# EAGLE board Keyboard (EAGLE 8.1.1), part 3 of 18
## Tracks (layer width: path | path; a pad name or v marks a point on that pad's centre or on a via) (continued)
S$1920 (continued)
  Bottom 0: 34.14,81.78 34.07,81.77
S$1921
  Bottom 0: 34.07,81.77 34,81.75
S$1922
  Bottom 0: 34,81.75 33.94,81.73
S$1923
  Bottom 0: 33.94,81.73 33.88,81.69
S$1924
  Bottom 0: 33.88,81.69 33.83,81.65
S$1925
  Bottom 0: 33.83,81.65 31.29,79.12
S$1926
  Bottom 0: 31.29,79.12 25.38,79.12
S$1927
  Bottom 0: 25.38,79.12 25.29,79.35
S$1928
  Bottom 0: 25.29,79.35 25.08,79.63
S$1929
  Bottom 0: 25.08,79.63 24.81,79.86
S$1930
  Bottom 0: 24.81,79.86 24.5,80.01
S$1931
  Bottom 0: 24.5,80.01 24.15,80.07
S$1932
  Bottom 0: 24.15,80.07 23.85,80.05
S$1933
  Bottom 0: 23.85,80.05 24.57,80.78
S$1934
  Bottom 0: 24.57,80.78 29.1,80.78
S$1935
  Bottom 0: 29.1,80.78 29.12,80.7
S$1936
  Bottom 0: 29.12,80.7 29.29,80.39
S$1937
  Bottom 0: 29.29,80.39 29.53,80.14
S$1938
  Bottom 0: 29.53,80.14 29.82,79.95
S$1939
  Bottom 0: 29.82,79.95 30.15,79.84
S$1940
  Bottom 0: 30.15,79.84 30.5,79.83
S$1941
  Bottom 0: 30.5,79.83 30.85,79.89
S$1942
  Bottom 0: 30.85,79.89 31.16,80.04
S$1943
  Bottom 0: 31.16,80.04 31.43,80.26
S$1944
  Bottom 0: 31.43,80.26 31.64,80.55
S$1945
  Bottom 0: 31.64,80.55 31.77,80.87
S$1946
  Bottom 0: 31.77,80.87 31.81,81.22
S$1947
  Bottom 0: 31.81,81.22 31.77,81.56
S$1948
  Bottom 0: 31.77,81.56 31.64,81.89
S$1949
  Bottom 0: 31.64,81.89 31.43,82.17
S$1950
  Bottom 0: 31.43,82.17 31.16,82.39
S$1951
  Bottom 0: 31.16,82.39 30.85,82.55
S$1952
  Bottom 0: 30.85,82.55 30.5,82.61
S$1953
  Bottom 0: 30.5,82.61 30.15,82.59
S$1954
  Bottom 0: 30.15,82.59 29.82,82.48
S$1955
  Bottom 0: 29.82,82.48 29.53,82.29
S$1956
  Bottom 0: 29.53,82.29 29.29,82.04
S$1957
  Bottom 0: 29.29,82.04 29.12,81.73
S$1958
  Bottom 0: 29.12,81.73 29.1,81.66
S$1959
  Bottom 0: 29.1,81.66 27.51,81.66
S$1960
  Bottom 0: 27.51,81.66 27.88,81.86
S$1961
  Bottom 0: 27.88,81.86 28.22,82.14
S$1962
  Bottom 0: 28.22,82.14 28.51,82.49
S$1963
  Bottom 0: 28.51,82.49 28.72,82.88
S$1964
  Bottom 0: 28.72,82.88 28.85,83.31
S$1965
  Bottom 0: 28.85,83.31 28.89,83.76
S$1966
  Bottom 0: 28.89,83.76 28.85,84.2
S$1967
  Bottom 0: 28.85,84.2 28.72,84.63
S$1968
  Bottom 0: 28.72,84.63 28.51,85.03
S$1969
  Bottom 0: 28.51,85.03 28.22,85.37
S$1970
  Bottom 0: 28.22,85.37 27.88,85.66
S$1971
  Bottom 0: 27.88,85.66 27.48,85.87
S$1972
  Bottom 0: 27.48,85.87 27.05,86
S$1973
  Bottom 0: 27.05,86 26.61,86.04
S$1974
  Bottom 0: 26.61,86.04 26.16,86
S$1975
  Bottom 0: 26.16,86 25.73,85.87
S$1976
  Bottom 0: 25.73,85.87 25.34,85.66
S$1977
  Bottom 0: 25.34,85.66 24.99,85.37
S$1978
  Bottom 0: 24.99,85.37 24.7,85.03
S$1979
  Bottom 0: 24.7,85.03 24.49,84.63
S$1980
  Bottom 0: 24.49,84.63 24.37,84.2
S$1981
  Bottom 0: 24.37,84.2 24.32,83.76
S$1982
  Bottom 0: 24.32,83.76 24.37,83.31
S$1983
  Bottom 0: 24.37,83.31 24.49,82.88
S$1984
  Bottom 0: 24.49,82.88 24.7,82.49
S$1985
  Bottom 0: 24.7,82.49 24.99,82.14
S$1986
  Bottom 0: 24.99,82.14 25.34,81.86
S$1987
  Bottom 0: 25.34,81.86 25.7,81.66
S$1988
  Bottom 0: 25.7,81.66 24.39,81.66
S$1989
  Bottom 0: 24.39,81.66 24.32,81.65
S$1990
  Bottom 0: 24.32,81.65 24.25,81.64
S$1991
  Bottom 0: 24.25,81.64 24.19,81.61
S$1992
  Bottom 0: 24.19,81.61 24.13,81.57
S$1993
  Bottom 0: 24.13,81.57 24.07,81.53
S$1994
  Bottom 0: 24.07,81.53 22.24,79.7
S$1995
  Bottom 0: 22.24,79.7 22.24,80.54
S$1996
  Bottom 0: 22.24,80.54 22.31,80.61
S$1997
  Bottom 0: 22.31,80.61 22.36,80.61
S$1998
  Bottom 0: 22.36,80.61 22.5,80.63
S$1999
  Bottom 0: 22.5,80.63 22.62,80.69
S$2000
  Bottom 0: 22.62,80.69 22.71,80.79
S$2001
  Bottom 0: 22.71,80.79 22.78,80.91
S$2002
  Bottom 0: 22.78,80.91 22.8,81.05
S$2003
  Bottom 0: 22.8,81.05 22.8,84.4
S$2004
  Bottom 0: 22.8,84.4 25.65,87.25
S$2005
  Bottom 0: 25.65,87.25 25.69,87.32
S$2006
  Bottom 0: 25.69,87.32 25.72,87.35
S$2007
  Bottom 0: 25.72,87.35 25.73,87.39
S$2008
  Bottom 0: 25.73,87.39 25.76,87.45
S$2009
  Bottom 0: 25.76,87.45 25.76,87.51
S$2010
  Bottom 0: 25.76,87.51 25.78,87.57
S$2011
  Bottom 0: 25.78,87.57 25.78,87.69
S$2012
  Bottom 0: 25.78,87.69 26.23,87.69
S$2013
  Bottom 0: 26.23,87.69 26.3,87.7
S$2014
  Bottom 0: 26.3,87.7 26.37,87.74
S$2015
  Bottom 0: 26.37,87.74 26.43,87.8
S$2016
  Bottom 0: 26.43,87.8 26.47,87.87
S$2017
  Bottom 0: 26.47,87.87 26.48,87.95
S$2018
  Bottom 0: 26.48,87.95 26.48,89.72
S$2019
  Bottom 0: 26.48,89.72 26.47,89.8
S$2020
  Bottom 0: 26.47,89.8 26.43,89.87
S$2021
  Bottom 0: 26.43,89.87 26.37,89.93
S$2022
  Bottom 0: 26.37,89.93 26.3,89.97
S$2023
  Bottom 0: 26.3,89.97 26.23,89.98
S$2024
  Bottom 0: 26.23,89.98 24.45,89.98
S$2025
  Bottom 0: 24.45,89.98 24.37,89.97
S$2026
  Bottom 0: 24.37,89.97 24.3,89.93
S$2027
  Bottom 0: 24.3,89.93 24.24,89.87
S$2028
  Bottom 0: 24.24,89.87 24.2,89.8
S$2029
  Bottom 0: 24.2,89.8 24.19,89.72
S$2030
  Bottom 0: 24.19,89.72 24.19,87.95
S$2031
  Bottom 0: 24.19,87.95 24.2,87.87
S$2032
  Bottom 0: 24.2,87.87 24.24,87.8
S$2033
  Bottom 0: 24.24,87.8 24.3,87.74
S$2034
  Bottom 0: 24.3,87.74 24.37,87.7
S$2035
  Bottom 0: 24.37,87.7 24.45,87.69
S$2036
  Bottom 0: 24.45,87.69 24.83,87.69
S$2037
  Bottom 0: 24.83,87.69 22.05,84.91
S$2038
  Bottom 0: 22.05,84.91 22,84.85
S$2039
  Bottom 0: 22,84.85 21.96,84.79
S$2040
  Bottom 0: 21.96,84.79 21.94,84.73
S$2041
  Bottom 0: 21.94,84.73 21.92,84.66
S$2042
  Bottom 0: 21.92,84.66 21.92,84.59
S$2043
  Bottom 0: 21.92,84.59 21.92,81.44
S$2044
  Bottom 0: 21.92,81.44 21.87,81.41
S$2045
  Bottom 0: 21.87,81.41 21.82,81.36
S$2046
  Bottom 0: 21.82,81.36 21.49,81.04
S$2047
  Bottom 0: 21.49,81.04 21.45,80.99
S$2048
  Bottom 0: 21.45,80.99 21.41,80.93
S$2049
  Bottom 0: 21.41,80.93 21.38,80.86
S$2050
  Bottom 0: 21.38,80.86 21.36,80.8
S$2051
  Bottom 0: 21.36,80.8 21.36,80.72
S$2052
  Bottom 0: 21.36,80.72 21.36,76.79
S$2053
  Bottom 0: 21.36,76.79 21.36,76.72
S$2054
  Bottom 0: 21.36,76.72 21.38,76.65
S$2055
  Bottom 0: 21.38,76.65 21.4,76.59
S$2056
  Bottom 0: 21.4,76.59 21.45,76.53
S$2057
  Bottom 0: 21.45,76.53 21.48,76.47
S$2058
  Bottom 0: 21.48,76.47 21.84,76.12
S$2059
  Bottom 0: 21.84,76.12 21.7,75.89
S$2060
  Bottom 0: 21.7,75.89 21.61,75.58
S$2061
  Bottom 0: 21.61,75.58 21.61,75.26
S$2062
  Bottom 0: 21.61,75.26 21.7,74.94
S$2063
  Bottom 0: 21.7,74.94 21.87,74.67
S$2064
  Bottom 0: 21.87,74.67 22.1,74.44
S$2065
  Bottom 0: 22.1,74.44 22.39,74.3
S$2066
  Bottom 0: 22.39,74.3 22.71,74.23
S$2067
  Bottom 0: 22.71,74.23 23.04,74.25
S$2068
  Bottom 0: 23.04,74.25 23.34,74.36
S$2069
  Bottom 0: 23.34,74.36 23.61,74.55
S$2070
  Bottom 0: 23.61,74.55 23.82,74.8
S$2071
  Bottom 0: 23.82,74.8 23.94,75.1
S$2072
  Bottom 0: 23.94,75.1 23.99,75.42
S$2073
  Bottom 0: 23.99,75.42 23.94,75.74
S$2074
  Bottom 0: 23.94,75.74 23.9,75.85
S$2075
  Bottom 0: 23.9,75.85 24.7,75.05
S$2076
  Bottom 0: 24.7,75.05 24.7,68.48
S$2077
  Bottom 0: 24.7,68.48 24.7,68.4
S$2078
  Bottom 0: 24.7,68.4 24.72,68.34
S$2079
  Bottom 0: 24.72,68.34 24.74,68.28
S$2080
  Bottom 0: 24.74,68.28 24.78,68.21
S$2081
  Bottom 0: 24.78,68.21 24.82,68.17
S$2082
  Bottom 0: 24.82,68.17 29.65,63.33
S$2083
  Bottom 0: 29.65,63.33 29.71,63.29
S$2084
  Bottom 0: 29.71,63.29 23.49,63.29
S$2085
  Bottom 0: 23.49,63.29 23.49,69.53
S$2086
  Bottom 0: 23.49,69.53 23.49,69.6
S$2087
  Bottom 0: 23.49,69.6 23.47,69.67
S$2088
  Bottom 0: 23.47,69.67 23.45,69.73
S$2089
  Bottom 0: 23.45,69.73 23.4,69.79
S$2090
  Bottom 0: 23.4,69.79 23.36,69.85
S$2091
  Bottom 0: 23.36,69.85 12.61,80.6
S$2092
  Bottom 0: 12.61,80.6 12.71,80.87
S$2093
  Bottom 0: 12.71,80.87 12.76,81.22
S$2094
  Bottom 0: 12.76,81.22 12.71,81.56
S$2095
  Bottom 0: 12.71,81.56 12.59,81.89
S$2096
  Bottom 0: 12.59,81.89 12.38,82.17
S$2097
  Bottom 0: 12.38,82.17 12.11,82.39
S$2098
  Bottom 0: 12.11,82.39 11.8,82.55
S$2099
  Bottom 0: 11.8,82.55 11.45,82.61
S$2100
  Bottom 0: 11.45,82.61 11.1,82.59
S$2101
  Bottom 0: 11.1,82.59 10.77,82.48
S$2102
  Bottom 0: 10.77,82.48 10.48,82.29
S$2103
  Bottom 0: 10.48,82.29 10.29,82.1
S$2104
  Bottom 0: 10.29,82.1 10.29,82.12
S$2105
  Bottom 0: 10.29,82.12 10.49,82.31
S$2106
  Bottom 0: 10.49,82.31 10.55,82.38
S$2107
  Bottom 0: 10.55,82.38 10.59,82.45
S$2108
  Bottom 0: 10.59,82.45 10.63,82.53
S$2109
  Bottom 0: 10.63,82.53 10.65,82.62
S$2110
  Bottom 0: 10.65,82.62 10.65,82.71
S$2111
  Bottom 0: 10.65,82.71 10.65,87.58
S$2112
  Bottom 0: 10.65,87.58 10.65,87.67
S$2113
  Bottom 0: 10.65,87.67 10.63,87.75
S$2114
  Bottom 0: 10.63,87.75 10.59,87.84
S$2115
  Bottom 0: 10.59,87.84 10.55,87.91
S$2116
  Bottom 0: 10.55,87.91 10.49,87.98
S$2117
  Bottom 0: 10.49,87.98 9.93,88.54
S$2118
  Bottom 0: 9.93,88.54 9.97,88.84
S$2119
  Bottom 0: 9.97,88.84 9.92,89.16
S$2120
  Bottom 0: 9.92,89.16 9.78,89.46
S$2121
  Bottom 0: 9.78,89.46 9.57,89.7
S$2122
  Bottom 0: 9.57,89.7 9.3,89.88
S$2123
  Bottom 0: 9.3,89.88 8.99,89.97
S$2124
  Bottom 0: 8.99,89.97 8.66,89.97
S$2125
  Bottom 0: 8.66,89.97 8.35,89.88
S$2126
  Bottom 0: 8.35,89.88 8.08,89.7
S$2127
  Bottom 0: 8.08,89.7 7.87,89.46
S$2128
  Bottom 0: 7.87,89.46 7.73,89.16
S$2129
  Bottom 0: 7.73,89.16 7.68,88.84
S$2130
  Bottom 0: 7.68,88.84 7.73,88.52
S$2131
  Bottom 0: 7.73,88.52 7.87,88.22
S$2132
  Bottom 0: 7.87,88.22 8.08,87.97
S$2133
  Bottom 0: 8.08,87.97 8.35,87.8
S$2134
  Bottom 0: 8.35,87.8 8.66,87.7
S$2135
  Bottom 0: 8.66,87.7 8.99,87.7
S$2136
  Bottom 0: 8.99,87.7 9.11,87.74
S$2137
  Bottom 0: 9.11,87.74 9.52,87.34
S$2138
  Bottom 0: 9.52,87.34 9.52,84.92
S$2139
  Bottom 0: 9.52,84.92 9.46,85.03
S$2140
  Bottom 0: 9.46,85.03 9.17,85.37
S$2141
  Bottom 0: 9.17,85.37 8.83,85.66
S$2142
  Bottom 0: 8.83,85.66 8.43,85.87
S$2143
  Bottom 0: 8.43,85.87 8,86
S$2144
  Bottom 0: 8,86 7.56,86.04
S$2145
  Bottom 0: 7.56,86.04 7.11,86
S$2146
  Bottom 0: 7.11,86 6.68,85.87
S$2147
  Bottom 0: 6.68,85.87 6.29,85.66
S$2148
  Bottom 0: 6.29,85.66 5.94,85.37
S$2149
  Bottom 0: 5.94,85.37 5.65,85.03
S$2150
  Bottom 0: 5.65,85.03 5.44,84.63
S$2151
  Bottom 0: 5.44,84.63 5.32,84.2
S$2152
  Bottom 0: 5.32,84.2 5.27,83.76
S$2153
  Bottom 0: 5.27,83.76 5.32,83.31
S$2154
  Bottom 0: 5.32,83.31 5.44,82.88
S$2155
  Bottom 0: 5.44,82.88 5.65,82.49
S$2156
  Bottom 0: 5.65,82.49 5.94,82.14
S$2157
  Bottom 0: 5.94,82.14 6.29,81.86
S$2158
  Bottom 0: 6.29,81.86 6.68,81.64
S$2159
  Bottom 0: 6.68,81.64 7.11,81.52
S$2160
  Bottom 0: 7.11,81.52 7.56,81.47
S$2161
  Bottom 0: 7.56,81.47 8,81.52
S$2162
  Bottom 0: 8,81.52 8.43,81.64
S$2163
  Bottom 0: 8.43,81.64 8.83,81.86
S$2164
  Bottom 0: 8.83,81.86 9.16,82.13
S$2165
  Bottom 0: 9.16,82.13 9.16,74.32
S$2166
  Bottom 0: 9.16,74.32 9.16,74.23
S$2167
  Bottom 0: 9.16,74.23 9.18,74.14
S$2168
  Bottom 0: 9.18,74.14 9.22,74.06
S$2169
  Bottom 0: 9.22,74.06 9.26,73.98
S$2170
  Bottom 0: 9.26,73.98 9.32,73.92
S$2171
  Bottom 0: 9.32,73.92 12.72,70.51
S$2172
  Bottom 0: 12.72,70.51 12.62,70.41
S$2173
  Bottom 0: 12.62,70.41 12.49,70.11
S$2174
  Bottom 0: 12.49,70.11 12.44,69.79
S$2175
  Bottom 0: 12.44,69.79 12.49,69.47
S$2176
  Bottom 0: 12.49,69.47 12.62,69.16
S$2177
  Bottom 0: 12.62,69.16 12.84,68.92
S$2178
  Bottom 0: 12.84,68.92 13.11,68.75
S$2179
  Bottom 0: 13.11,68.75 13.42,68.65
S$2180
  Bottom 0: 13.42,68.65 13.75,68.65
S$2181
  Bottom 0: 13.75,68.65 14.06,68.75
S$2182
  Bottom 0: 14.06,68.75 14.33,68.92
S$2183
  Bottom 0: 14.33,68.92 14.54,69.16
S$2184
  Bottom 0: 14.54,69.16 14.68,69.47
S$2185
  Bottom 0: 14.68,69.47 14.73,69.79
S$2186
  Bottom 0: 14.73,69.79 14.68,70.11
S$2187
  Bottom 0: 14.68,70.11 14.54,70.41
S$2188
  Bottom 0: 14.54,70.41 14.33,70.65
S$2189
  Bottom 0: 14.33,70.65 14.06,70.83
S$2190
  Bottom 0: 14.06,70.83 13.99,70.85
S$2191
  Bottom 0: 13.99,70.85 13.98,70.85
S$2192
  Bottom 0: 13.98,70.85 10.29,74.55
S$2193
  Bottom 0: 10.29,74.55 10.29,74.9
S$2194
  Bottom 0: 10.29,74.9 10.44,74.66
S$2195
  Bottom 0: 10.44,74.66 10.67,74.44
S$2196
  Bottom 0: 10.67,74.44 10.96,74.29
S$2197
  Bottom 0: 10.96,74.29 11.29,74.23
S$2198
  Bottom 0: 11.29,74.23 11.61,74.24
S$2199
  Bottom 0: 11.61,74.24 11.7,74.28
S$2200
  Bottom 0: 11.7,74.28 13.34,72.64
S$2201
  Bottom 0: 13.34,72.64 13.4,72.58
S$2202
  Bottom 0: 13.4,72.58 13.48,72.53
S$2203
  Bottom 0: 13.48,72.53 13.56,72.5
S$2204
  Bottom 0: 13.56,72.5 13.65,72.48
S$2205
  Bottom 0: 13.65,72.48 13.74,72.47
S$2206
  Bottom 0: 13.74,72.47 15.09,72.47
S$2207
  Bottom 0: 15.09,72.47 15.21,72.29
S$2208
  Bottom 0: 15.21,72.29 15.44,72.07
S$2209
  Bottom 0: 15.44,72.07 15.56,72.01
S$2210
  Bottom 0: 15.56,72.01 15.56,65.05
S$2211
  Bottom 0: 15.56,65.05 14.46,63.95
S$2212
  Bottom 0: 14.46,63.95 14.56,64.26
S$2213
  Bottom 0: 14.56,64.26 14.6,64.71
S$2214
  Bottom 0: 14.6,64.71 14.56,65.15
S$2215
  Bottom 0: 14.56,65.15 14.43,65.58
S$2216
  Bottom 0: 14.43,65.58 14.22,65.98
S$2217
  Bottom 0: 14.22,65.98 13.93,66.32
S$2218
  Bottom 0: 13.93,66.32 13.59,66.61
S$2219
  Bottom 0: 13.59,66.61 13.19,66.82
S$2220
  Bottom 0: 13.19,66.82 12.76,66.94
S$2221
  Bottom 0: 12.76,66.94 12.32,66.99
S$2222
  Bottom 0: 12.32,66.99 11.87,66.94
S$2223
  Bottom 0: 11.87,66.94 11.44,66.82
S$2224
  Bottom 0: 11.44,66.82 11.05,66.61
S$2225
  Bottom 0: 11.05,66.61 10.7,66.32
S$2226
  Bottom 0: 10.7,66.32 10.41,65.98
S$2227
  Bottom 0: 10.41,65.98 10.2,65.58
S$2228
  Bottom 0: 10.2,65.58 10.08,65.15
S$2229
  Bottom 0: 10.08,65.15 10.03,64.71
S$2230
  Bottom 0: 10.03,64.71 10.08,64.26
S$2231
  Bottom 0: 10.08,64.26 10.2,63.83
S$2232
  Bottom 0: 10.2,63.83 10.41,63.44
S$2233
  Bottom 0: 10.41,63.44 10.7,63.09
S$2234
  Bottom 0: 10.7,63.09 11.05,62.81
S$2235
  Bottom 0: 11.05,62.81 11.44,62.59
S$2236
  Bottom 0: 11.44,62.59 11.87,62.47
S$2237
  Bottom 0: 11.87,62.47 12.32,62.42
S$2238
  Bottom 0: 12.32,62.42 12.76,62.47
S$2239
  Bottom 0: 12.76,62.47 13.07,62.56
S$2240
  Bottom 0: 13.07,62.56 11.64,61.13
S$2241
  Bottom 0: 11.64,61.13 11.58,61.06
S$2242
  Bottom 0: 11.58,61.06 11.53,60.99
S$2243
  Bottom 0: 11.53,60.99 11.5,60.91
S$2244
  Bottom 0: 11.5,60.91 11.48,60.82
S$2245
  Bottom 0: 11.48,60.82 11.47,60.73
S$2246
  Bottom 0: 11.47,60.73 11.47,49.4
S$2247
  Bottom 0: 11.47,49.4 11.48,49.32
S$2248
  Bottom 0: 11.48,49.32 1.2,39.04
S$2249
  Bottom 0: 1.2,39.04 1.14,38.98
S$2250
  Bottom 0: 1.14,38.98 1.09,38.9
S$2251
  Bottom 0: 1.09,38.9 1.06,38.82
S$2252
  Bottom 0: 1.06,38.82 1.04,38.73
S$2253
  Bottom 0: 1.04,38.73 1.03,38.64
S$2254
  Bottom 0: 1.03,38.64 1.03,14.78
S$2255
  Bottom 0: 1.03,14.78 0.91,14.71
S$2256
  Bottom 0: 0.91,14.71 0.68,14.49
S$2257
  Bottom 0: 0.68,14.49 0.51,14.22
S$2258
  Bottom 0: 0.51,14.22 0.42,13.9
S$2259
  Bottom 0: 0.42,13.9 0.42,13.58
S$2260
  Bottom 0: 0.42,13.58 0.51,13.26
S$2261
  Bottom 0: 0.51,13.26 0.68,12.99
S$2262
  Bottom 0: 0.68,12.99 0.91,12.76
S$2263
  Bottom 0: 0.91,12.76 1.2,12.62
S$2264
  Bottom 0: 1.2,12.62 1.52,12.55
S$2265
  Bottom 0: 1.52,12.55 1.84,12.57
S$2266
  Bottom 0: 1.84,12.57 2.15,12.68
S$2267
  Bottom 0: 2.15,12.68 2.41,12.87
S$2268
  Bottom 0: 2.41,12.87 2.62,13.12
S$2269
  Bottom 0: 2.62,13.12 2.75,13.42
S$2270
  Bottom 0: 2.75,13.42 2.79,13.74
S$2271
  Bottom 0: 2.79,13.74 2.75,14.06
S$2272
  Bottom 0: 2.75,14.06 2.62,14.36
S$2273
  Bottom 0: 2.62,14.36 2.41,14.61
S$2274
  Bottom 0: 2.41,14.61 2.17,14.79
S$2275
  Bottom 0: 2.17,14.79 2.17,38.41
S$2276
  Bottom 0: 2.17,38.41 12.43,48.67
S$2277
  Bottom 0: 12.43,48.67 16.34,48.67
S$2278
  Bottom 0: 16.34,48.67 19.68,45.32
S$2279
  Bottom 0: 19.68,45.32 19.68,43.85
S$2280
  Bottom 0: 19.68,43.85 19.52,44.07
S$2281
  Bottom 0: 19.52,44.07 19.26,44.3
S$2282
  Bottom 0: 19.26,44.3 18.94,44.45
S$2283
  Bottom 0: 18.94,44.45 18.59,44.51
S$2284
  Bottom 0: 18.59,44.51 18.24,44.49
S$2285
  Bottom 0: 18.24,44.49 17.91,44.38
S$2286
  Bottom 0: 17.91,44.38 17.62,44.19
S$2287
  Bottom 0: 17.62,44.19 17.38,43.94
S$2288
  Bottom 0: 17.38,43.94 17.21,43.63
S$2289
  Bottom 0: 17.21,43.63 17.12,43.29
S$2290
  Bottom 0: 17.12,43.29 17.12,42.94
S$2291
  Bottom 0: 17.12,42.94 17.21,42.6
S$2292
  Bottom 0: 17.21,42.6 17.26,42.5
S$2293
  Bottom 0: 17.26,42.5 9.61,34.85
S$2294
  Bottom 0: 9.61,34.85 9.53,34.74
S$2295
  Bottom 0: 9.53,34.74 9.5,34.67
S$2296
  Bottom 0: 9.5,34.67 9.49,34.61
S$2297
  Bottom 0: 9.49,34.61 9.48,34.54
S$2298
  Bottom 0: 9.48,34.54 9.48,13.78
S$2299
  Bottom 0: 9.48,13.78 7.78,13.78
S$2300
  Bottom 0: 7.78,13.78 7.7,13.77
S$2301
  Bottom 0: 7.7,13.77 7.63,13.73
S$2302
  Bottom 0: 7.63,13.73 7.57,13.67
S$2303
  Bottom 0: 7.57,13.67 7.54,13.6
S$2304
  Bottom 0: 7.54,13.6 7.52,13.53
S$2305
  Bottom 0: 7.52,13.53 7.52,13.08
S$2306
  Bottom 0: 7.52,13.08 7.4,13.08
S$2307
  Bottom 0: 7.4,13.08 7.18,13.02
S$2308
  Bottom 0: 7.18,13.02 7.01,12.86
S$2309
  Bottom 0: 7.01,12.86 6.96,12.64
S$2310
  Bottom 0: 6.96,12.64 6.96,12.1
S$2311
  Bottom 0: 6.96,12.1 2.06,7.21
S$2312
  Bottom 0: 2.06,7.21 1.84,7.29
S$2313
  Bottom 0: 1.84,7.29 1.52,7.31
S$2314
  Bottom 0: 1.52,7.31 1.2,7.24
S$2315
  Bottom 0: 1.2,7.24 0.91,7.09
S$2316
  Bottom 0: 0.91,7.09 0.68,6.87
S$2317
  Bottom 0: 0.68,6.87 0.51,6.6
S$2318
  Bottom 0: 0.51,6.6 0.42,6.28
S$2319
  Bottom 0: 0.42,6.28 0.42,5.96
S$2320
  Bottom 0: 0.42,5.96 0.51,5.64
S$2321
  Bottom 0: 0.51,5.64 0.68,5.37
S$2322
  Bottom 0: 0.68,5.37 0.91,5.14
S$2323
  Bottom 0: 0.91,5.14 1.2,5
S$2324
  Bottom 0: 1.2,5 1.52,4.93
S$2325
  Bottom 0: 1.52,4.93 1.84,4.95
S$2326
  Bottom 0: 1.84,4.95 2.15,5.06
S$2327
  Bottom 0: 2.15,5.06 2.41,5.25
S$2328
  Bottom 0: 2.41,5.25 2.62,5.5
S$2329
  Bottom 0: 2.62,5.5 2.75,5.8
S$2330
  Bottom 0: 2.75,5.8 2.79,6.12
S$2331
  Bottom 0: 2.79,6.12 2.75,6.44
S$2332
  Bottom 0: 2.75,6.44 2.69,6.58
S$2333
  Bottom 0: 2.69,6.58 7.65,11.53
S$2334
  Bottom 0: 7.65,11.53 7.7,11.5
S$2335
  Bottom 0: 7.7,11.5 7.78,11.49
S$2336
  Bottom 0: 7.78,11.49 9.48,11.49
S$2337
  Bottom 0: 9.48,11.49 9.48,10.99
S$2338
  Bottom 0: 9.48,10.99 9.49,10.91
S$2339
  Bottom 0: 9.49,10.91 9.5,10.85
S$2340
  Bottom 0: 9.5,10.85 9.53,10.79
S$2341
  Bottom 0: 9.53,10.79 9.57,10.73
S$2342
  Bottom 0: 9.57,10.73 9.61,10.67
S$2343
  Bottom 0: 9.61,10.67 10.52,9.76
S$2344
  Bottom 0: 10.52,9.76 10.38,9.8
S$2345
  Bottom 0: 10.38,9.8 9.94,9.84
S$2346
  Bottom 0: 9.94,9.84 9.49,9.8
S$2347
  Bottom 0: 9.49,9.8 9.06,9.67
S$2348
  Bottom 0: 9.06,9.67 8.67,9.46
S$2349
  Bottom 0: 8.67,9.46 8.32,9.17
S$2350
  Bottom 0: 8.32,9.17 8.04,8.83
S$2351
  Bottom 0: 8.04,8.83 7.83,8.43
S$2352
  Bottom 0: 7.83,8.43 7.7,8
S$2353
  Bottom 0: 7.7,8 7.65,7.56
S$2354
  Bottom 0: 7.65,7.56 7.7,7.11
S$2355
  Bottom 0: 7.7,7.11 7.83,6.68
S$2356
  Bottom 0: 7.83,6.68 8.04,6.29
S$2357
  Bottom 0: 8.04,6.29 8.32,5.94
S$2358
  Bottom 0: 8.32,5.94 8.67,5.66
S$2359
  Bottom 0: 8.67,5.66 9.06,5.44
S$2360
  Bottom 0: 9.06,5.44 9.49,5.32
S$2361
  Bottom 0: 9.49,5.32 9.94,5.27
S$2362
  Bottom 0: 9.94,5.27 10.38,5.32
S$2363
  Bottom 0: 10.38,5.32 10.81,5.44
S$2364
  Bottom 0: 10.81,5.44 11.21,5.66
S$2365
  Bottom 0: 11.21,5.66 11.55,5.94
S$2366
  Bottom 0: 11.55,5.94 11.84,6.29
S$2367
  Bottom 0: 11.84,6.29 12.05,6.68
S$2368
  Bottom 0: 12.05,6.68 12.18,7.11
S$2369
  Bottom 0: 12.18,7.11 12.22,7.56
S$2370
  Bottom 0: 12.22,7.56 12.18,8
S$2371
  Bottom 0: 12.18,8 12.14,8.14
S$2372
  Bottom 0: 12.14,8.14 13.88,6.4
S$2373
  Bottom 0: 13.88,6.4 13.84,6.41
S$2374
  Bottom 0: 13.84,6.41 13.48,6.39
S$2375
  Bottom 0: 13.48,6.39 13.15,6.28
S$2376
  Bottom 0: 13.15,6.28 12.86,6.09
S$2377
  Bottom 0: 12.86,6.09 12.62,5.84
S$2378
  Bottom 0: 12.62,5.84 12.45,5.53
S$2379
  Bottom 0: 12.45,5.53 12.36,5.19
S$2380
  Bottom 0: 12.36,5.19 12.36,4.84
S$2381
  Bottom 0: 12.36,4.84 12.45,4.5
S$2382
  Bottom 0: 12.45,4.5 12.62,4.19
S$2383
  Bottom 0: 12.62,4.19 12.86,3.94
S$2384
  Bottom 0: 12.86,3.94 13.15,3.75
S$2385
  Bottom 0: 13.15,3.75 13.48,3.65
S$2386
  Bottom 0: 13.48,3.65 13.84,3.62
S$2387
  Bottom 0: 13.84,3.62 14.18,3.69
S$2388
  Bottom 0: 14.18,3.69 14.49,3.84
S$2389
  Bottom 0: 14.49,3.84 14.77,4.06
S$2390
  Bottom 0: 14.77,4.06 14.97,4.35
S$2391
  Bottom 0: 14.97,4.35 15.1,4.67
S$2392
  Bottom 0: 15.1,4.67 15.15,5.02
S$2393
  Bottom 0: 15.15,5.02 15.13,5.15
S$2394
  Bottom 0: 15.13,5.15 16.04,4.24
S$2395
  Bottom 0: 16.04,4.24 16.04,2.29
S$2396
  Bottom 0: 16.04,2.29 16.05,2.22
S$2397
  Bottom 0: 16.05,2.22 16.06,2.15
S$2398
  Bottom 0: 16.06,2.15 16.08,2.09
S$2399
  Bottom 0: 16.08,2.09 16.13,2.03
S$2400
  Bottom 0: 16.13,2.03 16.16,1.97
S$2401
  Bottom 0: 16.16,1.97 16.71,1.43
S$2402
  Bottom 0: 16.71,1.43 9.06,1.43
S$2403
  Bottom 0: 9.06,1.43 8.64,1.86
S$2404
  Bottom 0: 8.64,1.86 8.75,2.13
S$2405
  Bottom 0: 8.75,2.13 8.79,2.48
S$2406
  Bottom 0: 8.79,2.48 8.75,2.82
S$2407
  Bottom 0: 8.75,2.82 8.62,3.15
S$2408
  Bottom 0: 8.62,3.15 8.41,3.43
S$2409
  Bottom 0: 8.41,3.43 8.14,3.65
S$2410
  Bottom 0: 8.14,3.65 7.83,3.81
S$2411
  Bottom 0: 7.83,3.81 7.49,3.87
S$2412
  Bottom 0: 7.49,3.87 7.13,3.85
S$2413
  Bottom 0: 7.13,3.85 6.8,3.74
S$2414
  Bottom 0: 6.8,3.74 6.51,3.55
S$2415
  Bottom 0: 6.51,3.55 6.27,3.3
S$2416
  Bottom 0: 6.27,3.3 6.1,2.99
S$2417
  Bottom 0: 6.1,2.99 6.01,2.65
S$2418
  Bottom 0: 6.01,2.65 6.01,2.3
S$2419
  Bottom 0: 6.01,2.3 6.1,1.96
S$2420
  Bottom 0: 6.1,1.96 6.27,1.65
S$2421
  Bottom 0: 6.27,1.65 6.51,1.4
S$2422
  Bottom 0: 6.51,1.4 6.8,1.21
S$2423
  Bottom 0: 6.8,1.21 7.13,1.1
S$2424
  Bottom 0: 7.13,1.1 7.49,1.08
S$2425
  Bottom 0: 7.49,1.08 7.83,1.15
S$2426
  Bottom 0: 7.83,1.15 8.01,1.23
S$2427
  Bottom 0: 8.01,1.23 8.57,0.68
S$2428
  Bottom 0: 8.57,0.68 8.62,0.63
S$2429
  Bottom 0: 8.62,0.63 8.68,0.6
S$2430
  Bottom 0: 8.68,0.6 8.74,0.57
S$2431
  Bottom 0: 8.74,0.57 8.81,0.55
S$2432
  Bottom 0: 8.81,0.55 8.88,0.55
S$2433
  Bottom 0: 275.8,1.07 276.1,1.12
S$2434
  Bottom 0: 276.1,1.12 276.21,1.09
S$2435
  Bottom 0: 276.21,1.09 276.56,1.07
S$2436
  Bottom 0: 276.56,1.07 276.9,1.13
S$2437
  Bottom 0: 276.9,1.13 277.22,1.28
S$2438
  Bottom 0: 277.22,1.28 277.49,1.51
S$2439
  Bottom 0: 277.49,1.51 277.7,1.79
S$2440
  Bottom 0: 277.7,1.79 277.82,2.12
S$2441
  Bottom 0: 277.82,2.12 277.87,2.46
S$2442
  Bottom 0: 277.87,2.46 277.82,2.81
S$2443
  Bottom 0: 277.82,2.81 277.7,3.13
S$2444
  Bottom 0: 277.7,3.13 277.49,3.42
S$2445
  Bottom 0: 277.49,3.42 277.22,3.64
S$2446
  Bottom 0: 277.22,3.64 276.9,3.79
S$2447
  Bottom 0: 276.9,3.79 276.56,3.85
S$2448
  Bottom 0: 276.56,3.85 276.21,3.83
S$2449
  Bottom 0: 276.21,3.83 276.1,3.8
S$2450
  Bottom 0: 276.1,3.8 275.8,3.85
S$2451
  Bottom 0: 275.8,3.85 275.44,3.83
S$2452
  Bottom 0: 275.44,3.83 275.12,3.73
S$2453
  Bottom 0: 275.12,3.73 274.82,3.54
S$2454
  Bottom 0: 274.82,3.54 274.58,3.28
S$2455
  Bottom 0: 274.58,3.28 274.41,2.97
S$2456
  Bottom 0: 274.41,2.97 274.39,2.9
S$2457
  Bottom 0: 274.39,2.9 271.22,2.9
S$2458
  Bottom 0: 271.22,2.9 270.47,3.65
S$2459
  Bottom 0: 270.47,3.65 270.49,3.67
S$2460
  Bottom 0: 270.49,3.67 270.54,3.98
S$2461
  Bottom 0: 270.54,3.98 270.49,4.28
S$2462
  Bottom 0: 270.49,4.28 270.36,4.55
S$2463
  Bottom 0: 270.36,4.55 270.15,4.77
S$2464
  Bottom 0: 270.15,4.77 269.89,4.92
S$2465
  Bottom 0: 269.89,4.92 269.6,4.99
S$2466
  Bottom 0: 269.6,4.99 269.29,4.97
S$2467
  Bottom 0: 269.29,4.97 269.01,4.85
S$2468
  Bottom 0: 269.01,4.85 268.77,4.67
S$2469
  Bottom 0: 268.77,4.67 268.61,4.42
S$2470
  Bottom 0: 268.61,4.42 268.52,4.13
S$2471
  Bottom 0: 268.52,4.13 268.52,3.82
S$2472
  Bottom 0: 268.52,3.82 268.61,3.53
S$2473
  Bottom 0: 268.61,3.53 268.77,3.28
S$2474
  Bottom 0: 268.77,3.28 269.01,3.1
S$2475
  Bottom 0: 269.01,3.1 269.29,2.98
S$2476
  Bottom 0: 269.29,2.98 269.6,2.96
S$2477
  Bottom 0: 269.6,2.96 269.85,3.02
S$2478
  Bottom 0: 269.85,3.02 270.72,2.15
S$2479
  Bottom 0: 270.72,2.15 270.78,2.11
S$2480
  Bottom 0: 270.78,2.11 270.84,2.06
S$2481
  Bottom 0: 270.84,2.06 270.9,2.04
S$2482
  Bottom 0: 270.9,2.04 270.96,2.02
S$2483
  Bottom 0: 270.96,2.02 271.04,2.02
S$2484
  Bottom 0: 271.04,2.02 274.39,2.02
S$2485
  Bottom 0: 274.39,2.02 274.41,1.95
S$2486
  Bottom 0: 274.41,1.95 274.58,1.64
S$2487
  Bottom 0: 274.58,1.64 274.82,1.38
S$2488
  Bottom 0: 274.82,1.38 275.12,1.2
S$2489
  Bottom 0: 275.12,1.2 275.44,1.09
S$2490
  Bottom 0: 275.44,1.09 275.8,1.07
S$2491
  Bottom 0: 197.99,1.08 198.33,1.15
S$2492
  Bottom 0: 198.33,1.15 198.65,1.3
S$2493
  Bottom 0: 198.65,1.3 198.91,1.52
S$2494
  Bottom 0: 198.91,1.52 199.12,1.81
S$2495
  Bottom 0: 199.12,1.81 199.25,2.13
S$2496
  Bottom 0: 199.25,2.13 199.3,2.48
S$2497
  Bottom 0: 199.3,2.48 199.25,2.82
S$2498
  Bottom 0: 199.25,2.82 199.12,3.15
S$2499
  Bottom 0: 199.12,3.15 198.91,3.43
S$2500
  Bottom 0: 198.91,3.43 198.65,3.65
S$2501
  Bottom 0: 198.65,3.65 198.33,3.81
S$2502
  Bottom 0: 198.33,3.81 197.99,3.87
S$2503
  Bottom 0: 197.99,3.87 197.63,3.85
S$2504
  Bottom 0: 197.63,3.85 197.31,3.74
S$2505
  Bottom 0: 197.31,3.74 197.27,3.72
S$2506
  Bottom 0: 197.27,3.72 193.75,7.24
S$2507
  Bottom 0: 193.75,7.24 193.75,14.97
S$2508
  Bottom 0: 193.75,14.97 193.95,15.09
S$2509
  Bottom 0: 193.95,15.09 194.15,15.3
S$2510
  Bottom 0: 194.15,15.3 194.28,15.58
S$2511
  Bottom 0: 194.28,15.58 194.33,15.88
S$2512
  Bottom 0: 194.33,15.88 194.28,16.18
S$2513
  Bottom 0: 194.28,16.18 194.15,16.45
S$2514
  Bottom 0: 194.15,16.45 193.95,16.67
S$2515
  Bottom 0: 193.95,16.67 193.68,16.82
S$2516
  Bottom 0: 193.68,16.82 193.38,16.89
S$2517
  Bottom 0: 193.38,16.89 193.08,16.87
S$2518
  Bottom 0: 193.08,16.87 192.8,16.76
S$2519
  Bottom 0: 192.8,16.76 192.56,16.57
S$2520
  Bottom 0: 192.56,16.57 192.4,16.32
S$2521
  Bottom 0: 192.4,16.32 192.3,16.03
S$2522
  Bottom 0: 192.3,16.03 192.3,15.72
S$2523
  Bottom 0: 192.3,15.72 192.4,15.44
S$2524
  Bottom 0: 192.4,15.44 192.56,15.19
S$2525
  Bottom 0: 192.56,15.19 192.8,15
S$2526
  Bottom 0: 192.8,15 192.87,14.97
S$2527
  Bottom 0: 192.87,14.97 192.87,7.06
S$2528
  Bottom 0: 192.87,7.06 192.87,6.99
S$2529
  Bottom 0: 192.87,6.99 192.89,6.92
S$2530
  Bottom 0: 192.89,6.92 192.92,6.86
S$2531
  Bottom 0: 192.92,6.86 192.96,6.8
S$2532
  Bottom 0: 192.96,6.8 193,6.74
S$2533
  Bottom 0: 193,6.74 196.65,3.09
S$2534
  Bottom 0: 196.65,3.09 196.6,2.99
S$2535
  Bottom 0: 196.6,2.99 196.51,2.65
S$2536
  Bottom 0: 196.51,2.65 196.51,2.3
S$2537
  Bottom 0: 196.51,2.3 196.6,1.96
S$2538
  Bottom 0: 196.6,1.96 196.77,1.65
S$2539
  Bottom 0: 196.77,1.65 197.01,1.4
S$2540
  Bottom 0: 197.01,1.4 197.31,1.21
S$2541
  Bottom 0: 197.31,1.21 197.63,1.1
S$2542
  Bottom 0: 197.63,1.1 197.99,1.08
S$2543
  Bottom 0: 126.55,1.08 126.9,1.15
S$2544
  Bottom 0: 126.9,1.15 127.21,1.3
S$2545
  Bottom 0: 127.21,1.3 127.48,1.52
S$2546
  Bottom 0: 127.48,1.52 127.69,1.81
S$2547
  Bottom 0: 127.69,1.81 127.81,2.13
S$2548
  Bottom 0: 127.81,2.13 127.86,2.48
S$2549
  Bottom 0: 127.86,2.48 127.81,2.82
S$2550
  Bottom 0: 127.81,2.82 127.69,3.15
S$2551
  Bottom 0: 127.69,3.15 127.48,3.43
S$2552
  Bottom 0: 127.48,3.43 127.21,3.65
S$2553
  Bottom 0: 127.21,3.65 126.9,3.81
S$2554
  Bottom 0: 126.9,3.81 126.55,3.87
S$2555
  Bottom 0: 126.55,3.87 126.2,3.85
S$2556
  Bottom 0: 126.2,3.85 125.87,3.74
S$2557
  Bottom 0: 125.87,3.74 125.84,3.73
S$2558
  Bottom 0: 125.84,3.73 122.31,7.26
S$2559
  Bottom 0: 122.31,7.26 122.31,14.98
S$2560
  Bottom 0: 122.31,14.98 122.5,15.09
S$2561
  Bottom 0: 122.5,15.09 122.7,15.31
S$2562
  Bottom 0: 122.7,15.31 122.84,15.58
S$2563
  Bottom 0: 122.84,15.58 122.88,15.88
S$2564
  Bottom 0: 122.88,15.88 122.84,16.18
S$2565
  Bottom 0: 122.84,16.18 122.7,16.46
S$2566
  Bottom 0: 122.7,16.46 122.5,16.68
S$2567
  Bottom 0: 122.5,16.68 122.24,16.83
S$2568
  Bottom 0: 122.24,16.83 121.94,16.89
S$2569
  Bottom 0: 121.94,16.89 121.64,16.87
S$2570
  Bottom 0: 121.64,16.87 121.36,16.76
S$2571
  Bottom 0: 121.36,16.76 121.12,16.57
S$2572
  Bottom 0: 121.12,16.57 120.95,16.32
S$2573
  Bottom 0: 120.95,16.32 120.86,16.04
S$2574
  Bottom 0: 120.86,16.04 120.86,15.73
S$2575
  Bottom 0: 120.86,15.73 120.95,15.44
S$2576
  Bottom 0: 120.95,15.44 121.12,15.19
S$2577
  Bottom 0: 121.12,15.19 121.36,15
S$2578
  Bottom 0: 121.36,15 121.42,14.98
S$2579
  Bottom 0: 121.42,14.98 121.42,7.07
S$2580
  Bottom 0: 121.42,7.07 121.43,7
S$2581
  Bottom 0: 121.43,7 121.44,6.94
S$2582
  Bottom 0: 121.44,6.94 121.47,6.88
S$2583
  Bottom 0: 121.47,6.88 121.51,6.82
S$2584
  Bottom 0: 121.51,6.82 121.55,6.76
S$2585
  Bottom 0: 121.55,6.76 125.22,3.09
S$2586
  Bottom 0: 125.22,3.09 125.16,2.99
S$2587
  Bottom 0: 125.16,2.99 125.08,2.65
S$2588
  Bottom 0: 125.08,2.65 125.08,2.3
S$2589
  Bottom 0: 125.08,2.3 125.16,1.96
S$2590
  Bottom 0: 125.16,1.96 125.34,1.65
S$2591
  Bottom 0: 125.34,1.65 125.58,1.4
S$2592
  Bottom 0: 125.58,1.4 125.87,1.21
S$2593
  Bottom 0: 125.87,1.21 126.2,1.1
S$2594
  Bottom 0: 126.2,1.1 126.55,1.08
S$2595
  Bottom 0: 55.11,1.08 55.46,1.15
S$2596
  Bottom 0: 55.46,1.15 55.77,1.3
S$2597
  Bottom 0: 55.77,1.3 56.04,1.52
S$2598
  Bottom 0: 56.04,1.52 56.25,1.81
S$2599
  Bottom 0: 56.25,1.81 56.38,2.13
S$2600
  Bottom 0: 56.38,2.13 56.42,2.48
S$2601
  Bottom 0: 56.42,2.48 56.38,2.82
S$2602
  Bottom 0: 56.38,2.82 56.25,3.15
S$2603
  Bottom 0: 56.25,3.15 56.04,3.43
S$2604
  Bottom 0: 56.04,3.43 55.77,3.65
S$2605
  Bottom 0: 55.77,3.65 55.46,3.81
S$2606
  Bottom 0: 55.46,3.81 55.11,3.87
S$2607
  Bottom 0: 55.11,3.87 54.76,3.85
S$2608
  Bottom 0: 54.76,3.85 54.43,3.74
S$2609
  Bottom 0: 54.43,3.74 54.4,3.73
S$2610
  Bottom 0: 54.4,3.73 53.84,4.29
S$2611
  Bottom 0: 53.84,4.29 53.78,4.33
S$2612
  Bottom 0: 53.78,4.33 53.72,4.37
S$2613
  Bottom 0: 53.72,4.37 53.66,4.4
S$2614
  Bottom 0: 53.66,4.4 53.6,4.41
S$2615
  Bottom 0: 53.6,4.41 53.52,4.42
S$2616
  Bottom 0: 53.52,4.42 50.14,4.42
S$2617
  Bottom 0: 50.14,4.42 50.07,4.55
S$2618
  Bottom 0: 50.07,4.55 49.87,4.77
S$2619
  Bottom 0: 49.87,4.77 49.6,4.92
S$2620
  Bottom 0: 49.6,4.92 49.31,4.99
S$2621
  Bottom 0: 49.31,4.99 49,4.97
S$2622
  Bottom 0: 49,4.97 48.73,4.85
S$2623
  Bottom 0: 48.73,4.85 48.49,4.67
S$2624
  Bottom 0: 48.49,4.67 48.32,4.42
S$2625
  Bottom 0: 48.32,4.42 48.23,4.13
S$2626
  Bottom 0: 48.23,4.13 48.23,3.82
S$2627
  Bottom 0: 48.23,3.82 48.32,3.53
S$2628
  Bottom 0: 48.32,3.53 48.49,3.28
S$2629
  Bottom 0: 48.49,3.28 48.73,3.1
S$2630
  Bottom 0: 48.73,3.1 49,2.98
S$2631
  Bottom 0: 49,2.98 49.31,2.96
S$2632
  Bottom 0: 49.31,2.96 49.6,3.03
S$2633
  Bottom 0: 49.6,3.03 49.87,3.18
S$2634
  Bottom 0: 49.87,3.18 50.07,3.4
S$2635
  Bottom 0: 50.07,3.4 50.14,3.53
S$2636
  Bottom 0: 50.14,3.53 53.34,3.53
S$2637
  Bottom 0: 53.34,3.53 53.78,3.09
S$2638
  Bottom 0: 53.78,3.09 53.72,2.99
S$2639
  Bottom 0: 53.72,2.99 53.63,2.65
S$2640
  Bottom 0: 53.63,2.65 53.63,2.3
S$2641
  Bottom 0: 53.63,2.3 53.72,1.96
S$2642
  Bottom 0: 53.72,1.96 53.9,1.65
S$2643
  Bottom 0: 53.9,1.65 54.13,1.4
S$2644
  Bottom 0: 54.13,1.4 54.43,1.21
S$2645
  Bottom 0: 54.43,1.21 54.76,1.1
S$2646
  Bottom 0: 54.76,1.1 55.11,1.08
S$2647
  Bottom 0: 316.34,5.26 316.72,5.3
S$2648
  Bottom 0: 316.72,5.3 317.1,5.26
S$2649
  Bottom 0: 317.1,5.26 317.55,5.31
S$2650
  Bottom 0: 317.55,5.31 317.97,5.43
S$2651
  Bottom 0: 317.97,5.43 318.37,5.65
S$2652
  Bottom 0: 318.37,5.65 318.72,5.93
S$2653
  Bottom 0: 318.72,5.93 319,6.28
S$2654
  Bottom 0: 319,6.28 319.21,6.67
S$2655
  Bottom 0: 319.21,6.67 319.34,7.1
S$2656
  Bottom 0: 319.34,7.1 319.39,7.55
S$2657
  Bottom 0: 319.39,7.55 319.34,7.99
S$2658
  Bottom 0: 319.34,7.99 319.21,8.42
S$2659
  Bottom 0: 319.21,8.42 319,8.82
S$2660
  Bottom 0: 319,8.82 318.72,9.16
S$2661
  Bottom 0: 318.72,9.16 318.37,9.45
S$2662
  Bottom 0: 318.37,9.45 317.97,9.66
S$2663
  Bottom 0: 317.97,9.66 317.55,9.79
S$2664
  Bottom 0: 317.55,9.79 317.1,9.83
S$2665
  Bottom 0: 317.1,9.83 316.72,9.79
S$2666
  Bottom 0: 316.72,9.79 316.34,9.83
S$2667
  Bottom 0: 316.34,9.83 315.89,9.79
S$2668
  Bottom 0: 315.89,9.79 315.46,9.66
S$2669
  Bottom 0: 315.46,9.66 315.07,9.45
S$2670
  Bottom 0: 315.07,9.45 314.72,9.16
S$2671
  Bottom 0: 314.72,9.16 314.44,8.82
S$2672
  Bottom 0: 314.44,8.82 314.22,8.42
S$2673
  Bottom 0: 314.22,8.42 314.1,7.99
S$2674
  Bottom 0: 314.1,7.99 314.05,7.55
S$2675
  Bottom 0: 314.05,7.55 314.1,7.1
S$2676
  Bottom 0: 314.1,7.1 314.22,6.67
S$2677
  Bottom 0: 314.22,6.67 314.44,6.28
S$2678
  Bottom 0: 314.44,6.28 314.72,5.93
S$2679
  Bottom 0: 314.72,5.93 315.07,5.65
S$2680
  Bottom 0: 315.07,5.65 315.46,5.43
S$2681
  Bottom 0: 315.46,5.43 315.89,5.31
S$2682
  Bottom 0: 315.89,5.31 316.34,5.26
S$2683
  Bottom 0: 200.44,5.27 200.89,5.32
S$2684
  Bottom 0: 200.89,5.32 201.31,5.44
S$2685
  Bottom 0: 201.31,5.44 201.71,5.66
S$2686
  Bottom 0: 201.71,5.66 202.05,5.94
S$2687
  Bottom 0: 202.05,5.94 202.34,6.29
S$2688
  Bottom 0: 202.34,6.29 202.55,6.68
S$2689
  Bottom 0: 202.55,6.68 202.68,7.11
S$2690
  Bottom 0: 202.68,7.11 202.72,7.56
S$2691
  Bottom 0: 202.72,7.56 202.68,8
S$2692
  Bottom 0: 202.68,8 202.55,8.43
S$2693
  Bottom 0: 202.55,8.43 202.34,8.83
S$2694
  Bottom 0: 202.34,8.83 202.05,9.17
S$2695
  Bottom 0: 202.05,9.17 201.71,9.46
S$2696
  Bottom 0: 201.71,9.46 201.31,9.67
S$2697
  Bottom 0: 201.31,9.67 200.89,9.8
S$2698
  Bottom 0: 200.89,9.8 200.44,9.84
S$2699
  Bottom 0: 200.44,9.84 199.99,9.8
S$2700
  Bottom 0: 199.99,9.8 199.56,9.67
S$2701
  Bottom 0: 199.56,9.67 199.17,9.46
S$2702
  Bottom 0: 199.17,9.46 198.82,9.17
S$2703
  Bottom 0: 198.82,9.17 198.54,8.83
S$2704
  Bottom 0: 198.54,8.83 198.33,8.43
S$2705
  Bottom 0: 198.33,8.43 198.2,8
S$2706
  Bottom 0: 198.2,8 198.15,7.56
S$2707
  Bottom 0: 198.15,7.56 198.2,7.11
S$2708
  Bottom 0: 198.2,7.11 198.33,6.68
S$2709
  Bottom 0: 198.33,6.68 198.54,6.29
S$2710
  Bottom 0: 198.54,6.29 198.82,5.94
S$2711
  Bottom 0: 198.82,5.94 199.17,5.66
S$2712
  Bottom 0: 199.17,5.66 199.56,5.44
S$2713
  Bottom 0: 199.56,5.44 199.99,5.32
S$2714
  Bottom 0: 199.99,5.32 200.44,5.27
S$2715
  Bottom 0: 129,5.27 129.45,5.32
S$2716
  Bottom 0: 129.45,5.32 129.88,5.44
S$2717
  Bottom 0: 129.88,5.44 130.27,5.66
S$2718
  Bottom 0: 130.27,5.66 130.62,5.94
S$2719
  Bottom 0: 130.62,5.94 130.9,6.29
S$2720
  Bottom 0: 130.9,6.29 131.12,6.68
S$2721
  Bottom 0: 131.12,6.68 131.24,7.11
S$2722
  Bottom 0: 131.24,7.11 131.29,7.56
S$2723
  Bottom 0: 131.29,7.56 131.24,8
S$2724
  Bottom 0: 131.24,8 131.12,8.43
S$2725
  Bottom 0: 131.12,8.43 130.9,8.83
S$2726
  Bottom 0: 130.9,8.83 130.62,9.17
S$2727
  Bottom 0: 130.62,9.17 130.27,9.46
S$2728
  Bottom 0: 130.27,9.46 129.88,9.67
S$2729
  Bottom 0: 129.88,9.67 129.45,9.8
S$2730
  Bottom 0: 129.45,9.8 129,9.84
S$2731
  Bottom 0: 129,9.84 128.56,9.8
S$2732
  Bottom 0: 128.56,9.8 128.13,9.67
S$2733
  Bottom 0: 128.13,9.67 127.73,9.46
S$2734
  Bottom 0: 127.73,9.46 127.39,9.17
S$2735
  Bottom 0: 127.39,9.17 127.1,8.83
S$2736
  Bottom 0: 127.1,8.83 126.89,8.43
S$2737
  Bottom 0: 126.89,8.43 126.76,8
S$2738
  Bottom 0: 126.76,8 126.72,7.56
S$2739
  Bottom 0: 126.72,7.56 126.76,7.11
S$2740
  Bottom 0: 126.76,7.11 126.89,6.68
S$2741
  Bottom 0: 126.89,6.68 127.1,6.29
S$2742
  Bottom 0: 127.1,6.29 127.39,5.94
S$2743
  Bottom 0: 127.39,5.94 127.73,5.66
S$2744
  Bottom 0: 127.73,5.66 128.13,5.44
S$2745
  Bottom 0: 128.13,5.44 128.56,5.32
S$2746
  Bottom 0: 128.56,5.32 129,5.27
S$2747
  Bottom 0: 306.6,6.04 307.12,6.04
S$2748
  Bottom 0: 307.12,6.04 307.63,6.12
S$2749
  Bottom 0: 307.63,6.12 308.12,6.29
S$2750
  Bottom 0: 308.12,6.29 308.57,6.54
S$2751
  Bottom 0: 308.57,6.54 308.99,6.86
S$2752
  Bottom 0: 308.99,6.86 309.34,7.24
S$2753
  Bottom 0: 309.34,7.24 309.62,7.67
S$2754
  Bottom 0: 309.62,7.67 309.83,8.15
S$2755
  Bottom 0: 309.83,8.15 309.96,8.64
S$2756
  Bottom 0: 309.96,8.64 310,9.16
S$2757
  Bottom 0: 310,9.16 309.96,9.68
S$2758
  Bottom 0: 309.96,9.68 309.83,10.18
S$2759
  Bottom 0: 309.83,10.18 309.62,10.65
S$2760
  Bottom 0: 309.62,10.65 309.34,11.09
S$2761
  Bottom 0: 309.34,11.09 308.99,11.47
S$2762
  Bottom 0: 308.99,11.47 308.57,11.79
S$2763
  Bottom 0: 308.57,11.79 308.12,12.03
S$2764
  Bottom 0: 308.12,12.03 307.63,12.2
S$2765
  Bottom 0: 307.63,12.2 307.12,12.29
S$2766
  Bottom 0: 307.12,12.29 306.6,12.29
S$2767
  Bottom 0: 306.6,12.29 306.1,12.2
S$2768
  Bottom 0: 306.1,12.2 305.61,12.03
S$2769
  Bottom 0: 305.61,12.03 305.15,11.79
S$2770
  Bottom 0: 305.15,11.79 304.74,11.47
S$2771
  Bottom 0: 304.74,11.47 304.39,11.09
S$2772
  Bottom 0: 304.39,11.09 304.11,10.65
S$2773
  Bottom 0: 304.11,10.65 303.9,10.18
S$2774
  Bottom 0: 303.9,10.18 303.77,9.68
S$2775
  Bottom 0: 303.77,9.68 303.73,9.16
S$2776
  Bottom 0: 303.73,9.16 303.77,8.64
S$2777
  Bottom 0: 303.77,8.64 303.9,8.15
S$2778
  Bottom 0: 303.9,8.15 304.11,7.67
S$2779
  Bottom 0: 304.11,7.67 304.39,7.24
S$2780
  Bottom 0: 304.39,7.24 304.74,6.86
S$2781
  Bottom 0: 304.74,6.86 305.15,6.54
S$2782
  Bottom 0: 305.15,6.54 305.61,6.29
S$2783
  Bottom 0: 305.61,6.29 306.1,6.12
S$2784
  Bottom 0: 306.1,6.12 306.6,6.04
S$2785
  Bottom 0: 170.27,6.32 170.6,6.34
S$2786
  Bottom 0: 170.6,6.34 170.9,6.45
S$2787
  Bottom 0: 170.9,6.45 171.17,6.64
S$2788
  Bottom 0: 171.17,6.64 171.38,6.89
S$2789
  Bottom 0: 171.38,6.89 171.5,7.19
S$2790
  Bottom 0: 171.5,7.19 171.55,7.51
S$2791
  Bottom 0: 171.55,7.51 171.5,7.83
S$2792
  Bottom 0: 171.5,7.83 171.38,8.13
S$2793
  Bottom 0: 171.38,8.13 171.17,8.38
S$2794
  Bottom 0: 171.17,8.38 170.9,8.57
S$2795
  Bottom 0: 170.9,8.57 170.6,8.68
S$2796
  Bottom 0: 170.6,8.68 170.27,8.7
S$2797
  Bottom 0: 170.27,8.7 169.95,8.63
S$2798
  Bottom 0: 169.95,8.63 169.66,8.49
S$2799
  Bottom 0: 169.66,8.49 169.43,8.26
S$2800
  Bottom 0: 169.43,8.26 169.25,7.99
S$2801
  Bottom 0: 169.25,7.99 169.17,7.67
S$2802
  Bottom 0: 169.17,7.67 169.17,7.35
S$2803
  Bottom 0: 169.17,7.35 169.25,7.03
S$2804
  Bottom 0: 169.25,7.03 169.43,6.76
S$2805
  Bottom 0: 169.43,6.76 169.66,6.54
S$2806
  Bottom 0: 169.66,6.54 169.95,6.39
S$2807
  Bottom 0: 169.95,6.39 170.27,6.32
S$2808
  Bottom 0: 198.28,11.49 200.06,11.49
S$2809
  Bottom 0: 200.06,11.49 200.13,11.5
S$2810
  Bottom 0: 200.13,11.5 200.21,11.54
S$2811
  Bottom 0: 200.21,11.54 200.26,11.6
S$2812
  Bottom 0: 200.26,11.6 200.3,11.67
S$2813
  Bottom 0: 200.3,11.67 200.31,11.75
S$2814
  Bottom 0: 200.31,11.75 200.31,13.53
S$2815
  Bottom 0: 200.31,13.53 200.3,13.6
S$2816
  Bottom 0: 200.3,13.6 200.26,13.67
S$2817
  Bottom 0: 200.26,13.67 200.21,13.73
S$2818
  Bottom 0: 200.21,13.73 200.13,13.77
S$2819
  Bottom 0: 200.13,13.77 200.06,13.78
S$2820
  Bottom 0: 200.06,13.78 199.61,13.78
S$2821
  Bottom 0: 199.61,13.78 199.61,13.91
S$2822
  Bottom 0: 199.61,13.91 199.55,14.13
S$2823
  Bottom 0: 199.55,14.13 199.39,14.29
S$2824
  Bottom 0: 199.39,14.29 199.17,14.35
S$2825
  Bottom 0: 199.17,14.35 198.82,14.35
S$2826
  Bottom 0: 198.82,14.35 197.74,15.43
S$2827
  Bottom 0: 197.74,15.43 197.8,15.57
S$2828
  Bottom 0: 197.8,15.57 197.84,15.89
S$2829
  Bottom 0: 197.84,15.89 197.8,16.21
S$2830
  Bottom 0: 197.8,16.21 197.67,16.51
S$2831
  Bottom 0: 197.67,16.51 197.46,16.76
S$2832
  Bottom 0: 197.46,16.76 197.19,16.95
S$2833
  Bottom 0: 197.19,16.95 196.89,17.06
S$2834
  Bottom 0: 196.89,17.06 196.57,17.08
S$2835
  Bottom 0: 196.57,17.08 196.25,17.01
S$2836
  Bottom 0: 196.25,17.01 195.96,16.86
S$2837
  Bottom 0: 195.96,16.86 195.72,16.64
S$2838
  Bottom 0: 195.72,16.64 195.55,16.36
S$2839
  Bottom 0: 195.55,16.36 195.47,16.05
S$2840
  Bottom 0: 195.47,16.05 195.47,15.72
S$2841
  Bottom 0: 195.47,15.72 195.55,15.41
S$2842
  Bottom 0: 195.55,15.41 195.72,15.14
S$2843
  Bottom 0: 195.72,15.14 195.96,14.91
S$2844
  Bottom 0: 195.96,14.91 196.25,14.77
S$2845
  Bottom 0: 196.25,14.77 196.57,14.7
S$2846
  Bottom 0: 196.57,14.7 196.89,14.72
S$2847
  Bottom 0: 196.89,14.72 197.11,14.8
S$2848
  Bottom 0: 197.11,14.8 198.16,13.74
S$2849
  Bottom 0: 198.16,13.74 198.13,13.73
S$2850
  Bottom 0: 198.13,13.73 198.08,13.67
S$2851
  Bottom 0: 198.08,13.67 198.04,13.6
S$2852
  Bottom 0: 198.04,13.6 198.03,13.53
S$2853
  Bottom 0: 198.03,13.53 198.03,11.75
S$2854
  Bottom 0: 198.03,11.75 198.04,11.67
S$2855
  Bottom 0: 198.04,11.67 198.08,11.6
S$2856
  Bottom 0: 198.08,11.6 198.13,11.54
S$2857
  Bottom 0: 198.13,11.54 198.2,11.5
S$2858
  Bottom 0: 198.2,11.5 198.28,11.49
S$2859
  Bottom 0: 126.84,11.49 128.62,11.49
S$2860
  Bottom 0: 128.62,11.49 128.7,11.5
S$2861
  Bottom 0: 128.7,11.5 128.77,11.54
S$2862
  Bottom 0: 128.77,11.54 128.83,11.6
S$2863
  Bottom 0: 128.83,11.6 128.87,11.67
S$2864
  Bottom 0: 128.87,11.67 128.88,11.75
S$2865
  Bottom 0: 128.88,11.75 128.88,13.53
S$2866
  Bottom 0: 128.88,13.53 128.87,13.6
S$2867
  Bottom 0: 128.87,13.6 128.83,13.67
S$2868
  Bottom 0: 128.83,13.67 128.77,13.73
S$2869
  Bottom 0: 128.77,13.73 128.7,13.77
S$2870
  Bottom 0: 128.7,13.77 128.62,13.78
S$2871
  Bottom 0: 128.62,13.78 128.18,13.78
S$2872
  Bottom 0: 128.18,13.78 128.18,13.91
S$2873
  Bottom 0: 128.18,13.91 128.12,14.13
S$2874
  Bottom 0: 128.12,14.13 127.95,14.29
S$2875
  Bottom 0: 127.95,14.29 127.73,14.35
S$2876
  Bottom 0: 127.73,14.35 127.37,14.35
S$2877
  Bottom 0: 127.37,14.35 126.29,15.43
S$2878
  Bottom 0: 126.29,15.43 126.35,15.57
S$2879
  Bottom 0: 126.35,15.57 126.4,15.89
S$2880
  Bottom 0: 126.4,15.89 126.35,16.21
S$2881
  Bottom 0: 126.35,16.21 126.22,16.51
S$2882
  Bottom 0: 126.22,16.51 126.02,16.76
S$2883
  Bottom 0: 126.02,16.76 125.75,16.95
S$2884
  Bottom 0: 125.75,16.95 125.45,17.06
S$2885
  Bottom 0: 125.45,17.06 125.12,17.08
S$2886
  Bottom 0: 125.12,17.08 124.8,17.01
S$2887
  Bottom 0: 124.8,17.01 124.51,16.86
S$2888
  Bottom 0: 124.51,16.86 124.28,16.64
S$2889
  Bottom 0: 124.28,16.64 124.11,16.36
S$2890
  Bottom 0: 124.11,16.36 124.02,16.05
S$2891
  Bottom 0: 124.02,16.05 124.02,15.72
S$2892
  Bottom 0: 124.02,15.72 124.11,15.41
S$2893
  Bottom 0: 124.11,15.41 124.28,15.14
S$2894
  Bottom 0: 124.28,15.14 124.51,14.91
S$2895
  Bottom 0: 124.51,14.91 124.8,14.77
S$2896
  Bottom 0: 124.8,14.77 125.12,14.7
S$2897
  Bottom 0: 125.12,14.7 125.45,14.72
S$2898
  Bottom 0: 125.45,14.72 125.67,14.8
S$2899
  Bottom 0: 125.67,14.8 126.72,13.74
S$2900
  Bottom 0: 126.72,13.74 126.69,13.73
S$2901
  Bottom 0: 126.69,13.73 126.64,13.67
S$2902
  Bottom 0: 126.64,13.67 126.6,13.6
S$2903
  Bottom 0: 126.6,13.6 126.59,13.53
S$2904
  Bottom 0: 126.59,13.53 126.59,11.75
S$2905
  Bottom 0: 126.59,11.75 126.6,11.67
S$2906
  Bottom 0: 126.6,11.67 126.64,11.6
S$2907
  Bottom 0: 126.64,11.6 126.69,11.54
S$2908
  Bottom 0: 126.69,11.54 126.77,11.5
S$2909
  Bottom 0: 126.77,11.5 126.84,11.49
S$2910
  Bottom 0: 181.31,20.14 181.66,20.2
S$2911
  Bottom 0: 181.66,20.2 181.97,20.35
S$2912
  Bottom 0: 181.97,20.35 182.24,20.57
S$2913
  Bottom 0: 182.24,20.57 182.45,20.86
S$2914
  Bottom 0: 182.45,20.86 182.58,21.18
S$2915
  Bottom 0: 182.58,21.18 182.62,21.53
S$2916
  Bottom 0: 182.62,21.53 182.58,21.87
S$2917
  Bottom 0: 182.58,21.87 182.45,22.2
S$2918
  Bottom 0: 182.45,22.2 182.24,22.48
S$2919
  Bottom 0: 182.24,22.48 181.97,22.7
S$2920
  Bottom 0: 181.97,22.7 181.66,22.86
S$2921
  Bottom 0: 181.66,22.86 181.31,22.92
S$2922
  Bottom 0: 181.31,22.92 180.96,22.9
S$2923
  Bottom 0: 180.96,22.9 180.63,22.79
S$2924
  Bottom 0: 180.63,22.79 180.34,22.6
S$2925
  Bottom 0: 180.34,22.6 180.1,22.35
S$2926
  Bottom 0: 180.1,22.35 179.92,22.04
S$2927
  Bottom 0: 179.92,22.04 179.84,21.7
S$2928
  Bottom 0: 179.84,21.7 179.84,21.35
S$2929
  Bottom 0: 179.84,21.35 179.92,21.01
S$2930
  Bottom 0: 179.92,21.01 180.1,20.7
S$2931
  Bottom 0: 180.1,20.7 180.34,20.45
S$2932
  Bottom 0: 180.34,20.45 180.63,20.26
S$2933
  Bottom 0: 180.63,20.26 180.96,20.16
S$2934
  Bottom 0: 180.96,20.16 181.31,20.14
S$2935
  Bottom 0: 174.33,22.02 174.63,22.09
S$2936
  Bottom 0: 174.63,22.09 174.89,22.24
S$2937
  Bottom 0: 174.89,22.24 175.09,22.46
S$2938
  Bottom 0: 175.09,22.46 175.22,22.73
S$2939
  Bottom 0: 175.22,22.73 175.27,23.03
S$2940
  Bottom 0: 175.27,23.03 175.22,23.33
S$2941
  Bottom 0: 175.22,23.33 175.09,23.6
S$2942
  Bottom 0: 175.09,23.6 174.89,23.82
S$2943
  Bottom 0: 174.89,23.82 174.63,23.98
S$2944
  Bottom 0: 174.63,23.98 174.33,24.04
S$2945
  Bottom 0: 174.33,24.04 174.03,24.02
S$2946
  Bottom 0: 174.03,24.02 173.75,23.91
S$2947
  Bottom 0: 173.75,23.91 173.51,23.72
S$2948
  Bottom 0: 173.51,23.72 173.34,23.47
S$2949
  Bottom 0: 173.34,23.47 173.25,23.18
S$2950
  Bottom 0: 173.25,23.18 173.25,22.88
S$2951
  Bottom 0: 173.25,22.88 173.34,22.59
S$2952
  Bottom 0: 173.34,22.59 173.51,22.34
S$2953
  Bottom 0: 173.51,22.34 173.75,22.15
S$2954
  Bottom 0: 173.75,22.15 174.03,22.04
S$2955
  Bottom 0: 174.03,22.04 174.33,22.02
S$2956
  Bottom 0: 136.23,22.02 136.52,22.09
S$2957
  Bottom 0: 136.52,22.09 136.79,22.24
S$2958
  Bottom 0: 136.79,22.24 136.99,22.46
S$2959
  Bottom 0: 136.99,22.46 137.12,22.73
S$2960
  Bottom 0: 137.12,22.73 137.17,23.03
S$2961
  Bottom 0: 137.17,23.03 137.12,23.33
S$2962
  Bottom 0: 137.12,23.33 136.99,23.6
S$2963
  Bottom 0: 136.99,23.6 136.79,23.82
S$2964
  Bottom 0: 136.79,23.82 136.52,23.98
S$2965
  Bottom 0: 136.52,23.98 136.23,24.04
S$2966
  Bottom 0: 136.23,24.04 135.92,24.02
S$2967
  Bottom 0: 135.92,24.02 135.64,23.91
S$2968
  Bottom 0: 135.64,23.91 135.41,23.72
S$2969
  Bottom 0: 135.41,23.72 135.24,23.47
S$2970
  Bottom 0: 135.24,23.47 135.15,23.18
S$2971
  Bottom 0: 135.15,23.18 135.15,22.88
S$2972
  Bottom 0: 135.15,22.88 135.24,22.59
S$2973
  Bottom 0: 135.24,22.59 135.41,22.34
S$2974
  Bottom 0: 135.41,22.34 135.64,22.15
S$2975
  Bottom 0: 135.64,22.15 135.92,22.04
S$2976
  Bottom 0: 135.92,22.04 136.23,22.02
S$2977
  Bottom 0: 183.77,24.32 184.21,24.37
S$2978
  Bottom 0: 184.21,24.37 184.64,24.49
S$2979
  Bottom 0: 184.64,24.49 185.04,24.71
S$2980
  Bottom 0: 185.04,24.71 185.38,24.99
S$2981
  Bottom 0: 185.38,24.99 185.67,25.34
S$2982
  Bottom 0: 185.67,25.34 185.88,25.73
S$2983
  Bottom 0: 185.88,25.73 186.01,26.16
S$2984
  Bottom 0: 186.01,26.16 186.05,26.61
S$2985
  Bottom 0: 186.05,26.61 186.01,27.05
S$2986
  Bottom 0: 186.01,27.05 185.88,27.48
S$2987
  Bottom 0: 185.88,27.48 185.67,27.88
S$2988
  Bottom 0: 185.67,27.88 185.38,28.22
S$2989
  Bottom 0: 185.38,28.22 185.04,28.51
S$2990
  Bottom 0: 185.04,28.51 184.64,28.72
S$2991
  Bottom 0: 184.64,28.72 184.21,28.85
S$2992
  Bottom 0: 184.21,28.85 183.77,28.89
S$2993
  Bottom 0: 183.77,28.89 183.32,28.85
S$2994
  Bottom 0: 183.32,28.85 182.89,28.72
S$2995
  Bottom 0: 182.89,28.72 182.5,28.51
S$2996
  Bottom 0: 182.5,28.51 182.15,28.22
S$2997
  Bottom 0: 182.15,28.22 181.87,27.88
S$2998
  Bottom 0: 181.87,27.88 181.65,27.48
S$2999
  Bottom 0: 181.65,27.48 181.53,27.05
S$3000
  Bottom 0: 181.53,27.05 181.48,26.61
S$3001
  Bottom 0: 181.48,26.61 181.53,26.16
S$3002
  Bottom 0: 181.53,26.16 181.65,25.73
S$3003
  Bottom 0: 181.65,25.73 181.87,25.34
S$3004
  Bottom 0: 181.87,25.34 182.15,24.99
S$3005
  Bottom 0: 182.15,24.99 182.5,24.71
S$3006
  Bottom 0: 182.5,24.71 182.89,24.49
S$3007
  Bottom 0: 182.89,24.49 183.32,24.37
S$3008
  Bottom 0: 183.32,24.37 183.77,24.32
S$3009
  Bottom 0: 126.62,24.32 127.06,24.37
S$3010
  Bottom 0: 127.06,24.37 127.49,24.49
S$3011
  Bottom 0: 127.49,24.49 127.89,24.71
S$3012
  Bottom 0: 127.89,24.71 128.23,24.99
S$3013
  Bottom 0: 128.23,24.99 128.52,25.34
S$3014
  Bottom 0: 128.52,25.34 128.73,25.73
S$3015
  Bottom 0: 128.73,25.73 128.85,26.16
S$3016
  Bottom 0: 128.85,26.16 128.9,26.61
S$3017
  Bottom 0: 128.9,26.61 128.85,27.05
S$3018
  Bottom 0: 128.85,27.05 128.73,27.48
S$3019
  Bottom 0: 128.73,27.48 128.52,27.88
S$3020
  Bottom 0: 128.52,27.88 128.23,28.22
S$3021
  Bottom 0: 128.23,28.22 127.89,28.51
S$3022
  Bottom 0: 127.89,28.51 127.49,28.72
S$3023
  Bottom 0: 127.49,28.72 127.06,28.85
S$3024
  Bottom 0: 127.06,28.85 126.62,28.89
S$3025
  Bottom 0: 126.62,28.89 126.17,28.85
S$3026
  Bottom 0: 126.17,28.85 125.74,28.72
S$3027
  Bottom 0: 125.74,28.72 125.35,28.51
S$3028
  Bottom 0: 125.35,28.51 125,28.22
S$3029
  Bottom 0: 125,28.22 124.72,27.88
S$3030
  Bottom 0: 124.72,27.88 124.5,27.48
S$3031
  Bottom 0: 124.5,27.48 124.37,27.05
S$3032
  Bottom 0: 124.37,27.05 124.33,26.61
S$3033
  Bottom 0: 124.33,26.61 124.37,26.16
S$3034
  Bottom 0: 124.37,26.16 124.5,25.73
S$3035
  Bottom 0: 124.5,25.73 124.72,25.34
S$3036
  Bottom 0: 124.72,25.34 125,24.99
S$3037
  Bottom 0: 125,24.99 125.35,24.71
S$3038
  Bottom 0: 125.35,24.71 125.74,24.49
S$3039
  Bottom 0: 125.74,24.49 126.17,24.37
S$3040
  Bottom 0: 126.17,24.37 126.62,24.32
S$3041
  Bottom 0: 9.62,36.13 9.94,36.15
S$3042
  Bottom 0: 9.94,36.15 10.25,36.25
S$3043
  Bottom 0: 10.25,36.25 10.51,36.44
S$3044
  Bottom 0: 10.51,36.44 10.72,36.7
S$3045
  Bottom 0: 10.72,36.7 10.85,36.99
S$3046
  Bottom 0: 10.85,36.99 10.89,37.31
S$3047
  Bottom 0: 10.89,37.31 10.85,37.63
S$3048
  Bottom 0: 10.85,37.63 10.72,37.94
S$3049
  Bottom 0: 10.72,37.94 10.51,38.19
S$3050
  Bottom 0: 10.51,38.19 10.25,38.38
S$3051
  Bottom 0: 10.25,38.38 9.94,38.48
S$3052
  Bottom 0: 9.94,38.48 9.62,38.5
S$3053
  Bottom 0: 9.62,38.5 9.3,38.44
S$3054
  Bottom 0: 9.3,38.44 9.01,38.29
S$3055
  Bottom 0: 9.01,38.29 8.78,38.07
S$3056
  Bottom 0: 8.78,38.07 8.6,37.79
S$3057
  Bottom 0: 8.6,37.79 8.51,37.48
S$3058
  Bottom 0: 8.51,37.48 8.51,37.15
S$3059
  Bottom 0: 8.51,37.15 8.6,36.84
S$3060
  Bottom 0: 8.6,36.84 8.78,36.56
S$3061
  Bottom 0: 8.78,36.56 9.01,36.34
S$3062
  Bottom 0: 9.01,36.34 9.3,36.19
S$3063
  Bottom 0: 9.3,36.19 9.62,36.13
S$3064
  Bottom 0: 12.24,39.19 12.59,39.25
S$3065
  Bottom 0: 12.59,39.25 12.91,39.4
S$3066
  Bottom 0: 12.91,39.4 13.18,39.62
S$3067
  Bottom 0: 13.18,39.62 13.38,39.91
S$3068
  Bottom 0: 13.38,39.91 13.51,40.23
S$3069
  Bottom 0: 13.51,40.23 13.56,40.58
S$3070
  Bottom 0: 13.56,40.58 13.51,40.92
S$3071
  Bottom 0: 13.51,40.92 13.38,41.25
S$3072
  Bottom 0: 13.38,41.25 13.18,41.53
S$3073
  Bottom 0: 13.18,41.53 12.91,41.76
S$3074
  Bottom 0: 12.91,41.76 12.59,41.91
S$3075
  Bottom 0: 12.59,41.91 12.24,41.97
S$3076
  Bottom 0: 12.24,41.97 11.89,41.95
S$3077
  Bottom 0: 11.89,41.95 11.56,41.84
S$3078
  Bottom 0: 11.56,41.84 11.27,41.65
S$3079
  Bottom 0: 11.27,41.65 11.03,41.4
S$3080
  Bottom 0: 11.03,41.4 10.86,41.09
S$3081
  Bottom 0: 10.86,41.09 10.77,40.75
S$3082
  Bottom 0: 10.77,40.75 10.77,40.4
S$3083
  Bottom 0: 10.77,40.4 10.86,40.06
S$3084
  Bottom 0: 10.86,40.06 11.03,39.75
S$3085
  Bottom 0: 11.03,39.75 11.27,39.5
S$3086
  Bottom 0: 11.27,39.5 11.56,39.31
S$3087
  Bottom 0: 11.56,39.31 11.89,39.2
S$3088
  Bottom 0: 11.89,39.2 12.24,39.19
S$3089
  Bottom 0: 14.7,43.37 15.15,43.42
S$3090
  Bottom 0: 15.15,43.42 15.57,43.54
S$3091
  Bottom 0: 15.57,43.54 15.97,43.76
S$3092
  Bottom 0: 15.97,43.76 16.31,44.04
S$3093
  Bottom 0: 16.31,44.04 16.6,44.39
S$3094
